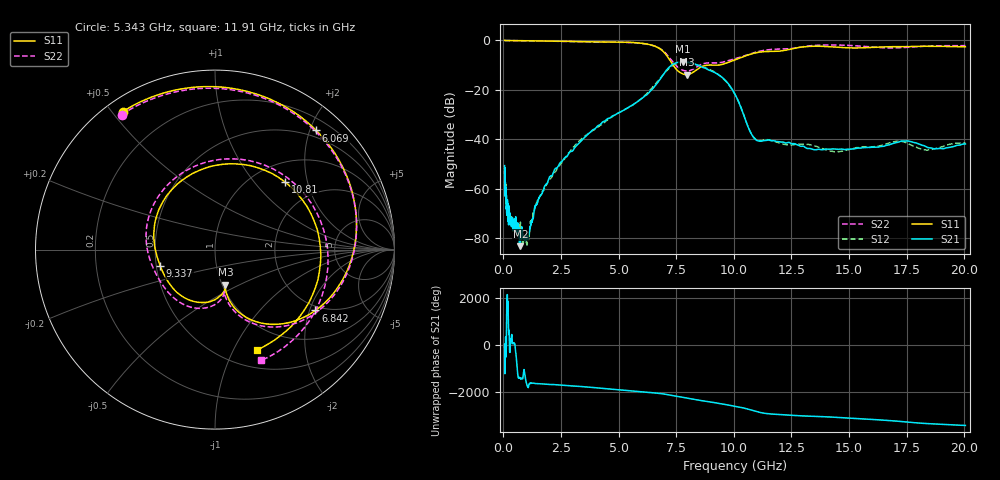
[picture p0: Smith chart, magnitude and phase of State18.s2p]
# Hz S DB R 50
!freq MagS11 AngS11 MagS21 AngS21 MagS12 AngS12 MagS22 AngS22
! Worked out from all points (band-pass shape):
!   1601 points, 50 MHz to 20.05 GHz, reference 50 ohm
!   highest |S21| = -8.56 dB at 7.8 GHz (marker M1); lowest = -83.1 dB at 733.7 MHz (marker M2)
!   |S21| within 3 dB of the highest: 7.113 GHz to 8.83 GHz (1.717 GHz wide, 21.5 % of centre)
!   lowest |S11| = -13.8 dB at 7.948 GHz (marker M3), VSWR 1.51, Z = 51.8 - j21.1 ohm
!   |S11| at or under -10 dB: 7.367 GHz to 8.825 GHz (1.458 GHz wide, 18 % of centre); 9.135 GHz to 9.224 GHz (89.03 MHz wide, 0.97 % of centre)
!   |S22| runs from -12.3 to 0.0 dB; largest |S21 - S12| = 0.022
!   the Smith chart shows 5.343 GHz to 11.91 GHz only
!   S11 on the Smith chart (normalised r, x): 5.343 GHz: 0.05, +0.53; 6.069 GHz: 0.38, +2.10; 6.842 GHz: 1.85, -2.20; 9.337 GHz: 0.53, -0.11; 10.81 GHz: 1.38, +1.47; 11.91 GHz: 0.71, -1.25
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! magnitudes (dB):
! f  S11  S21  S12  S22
! 50 MHz  0.0  -50.6  -58.8  0.0
! 64.27 MHz  0.0  -57.4  -56.2  0.0
! 75.5 MHz  0.0  -62.2  -60.8  0.0
! 89.7 MHz  0.0  -60.6  -58.0  0.0
! 101.1 MHz  0.0  -60.5  -65.7  0.0
! 135.9 MHz  0.0  -67.2  -66.8  0.0
! 369.6 MHz  0.0  -72.5  -71.8  0.0
! 531.6 MHz  -0.1  -71.2  -75.9  -0.1
! 733.7 MHz  -0.1  -83.1  -73.6  -0.1
! 1.005 GHz  -0.1  -78.6  -81.4  -0.1
! 2.722 GHz  -0.3  -47.1  -46.9  -0.4
! 5.343 GHz  -0.7  -27.5  -27.5  -0.8
! 6.069 GHz  -1.2  -22.9  -22.8  -1.3
! 6.842 GHz  -3.7  -15.1  -14.8  -3.6
! 7.402 GHz  -10.4  -9.4  -9.9  -9.2
! 7.8 GHz  -13.6  -8.6  -8.9  -12.1
! 7.948 GHz  -13.8  -8.7  -9.0  -12.3
! 9.337 GHz  -9.9  -13.9  -13.8  -9.0
! 9.951 GHz  -8.2  -20.1  -20.2  -7.6
! 10.81 GHz  -5.3  -38.5  -38.4  -5.1
! 11.91 GHz  -4.3  -40.8  -41.2  -3.5
! 20.05 GHz  -2.5  -41.8  -41.4  -2.1
